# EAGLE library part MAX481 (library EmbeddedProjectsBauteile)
RS422/485-Transceiver
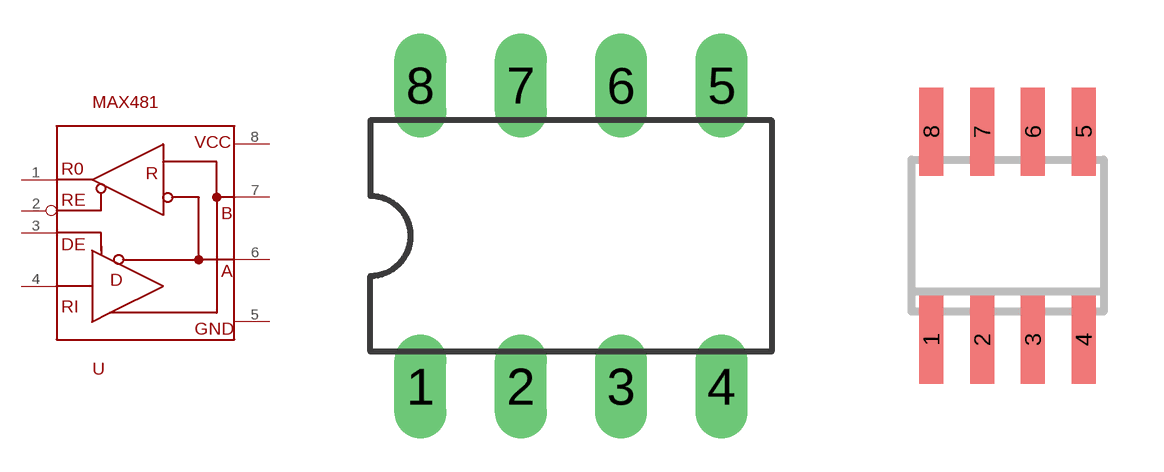
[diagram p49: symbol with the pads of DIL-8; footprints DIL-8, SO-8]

Designator prefix -

## MAX481ECPA  [DIL-8]
1  P$1  out
2  P$2  in
3  P$3  in
4  P$4  in
5  P$5  pwr
6  P$6
7  P$7
8  P$8  pwr

## MAX481CSA  [SO-8]
Pads as for DIL-8

## Footprint DIL-8 (pad centres in mm)
DIL
drill 0.813 long: 1 -3.81,-3.81; 2 -1.27,-3.81; 3 1.27,-3.81; 4 3.81,-3.81; 5 3.81,3.81; 6 1.27,3.81; 7 -1.27,3.81; 8 -3.81,3.81

## Footprint SO-8 (pad centres in mm)
smd 0.6 x 2.2: 1 -1.905,-2.6; 2 -0.635,-2.6; 3 0.635,-2.6; 4 1.905,-2.6; 5 1.905,2.6; 6 0.635,2.6; 7 -0.635,2.6; 8 -1.905,2.6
